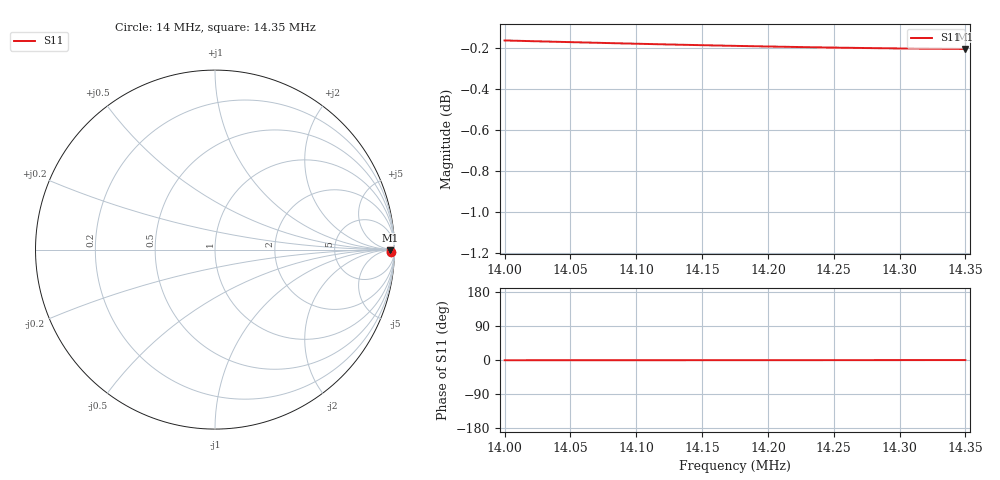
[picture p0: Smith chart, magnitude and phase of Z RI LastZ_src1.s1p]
! EZNEC Pro/4 beta ver. A6.0
! 5/17/2015 1:03:51 PM
! Back yard dipole
! Source 1
# MHZ Z RI R 50
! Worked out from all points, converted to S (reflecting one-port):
!   15 points, 14 MHz to 14.35 MHz, reference 50 ohm
!   lowest |S11| = -0.2 dB at 14.35 MHz (marker M1), VSWR 83.78, Z = 4.12e+03 - j550 ohm
!   phase of S11 starts at -1 deg and turns +0 deg over the sweep
14  79.16 -45.07
14.025  79.39 -42.64
14.05  79.62 -40.2
14.075  79.84 -37.76
14.1  80.07 -35.33
14.125  80.3 -32.89
14.15  80.52 -30.46
14.175  80.75 -28.02
14.2  80.97 -25.59
14.225  81.19 -23.16
14.25  81.42 -20.73
14.275  81.64 -18.3
14.3  81.86 -15.86
14.325  82.09 -13.43
14.35  82.31 -11
